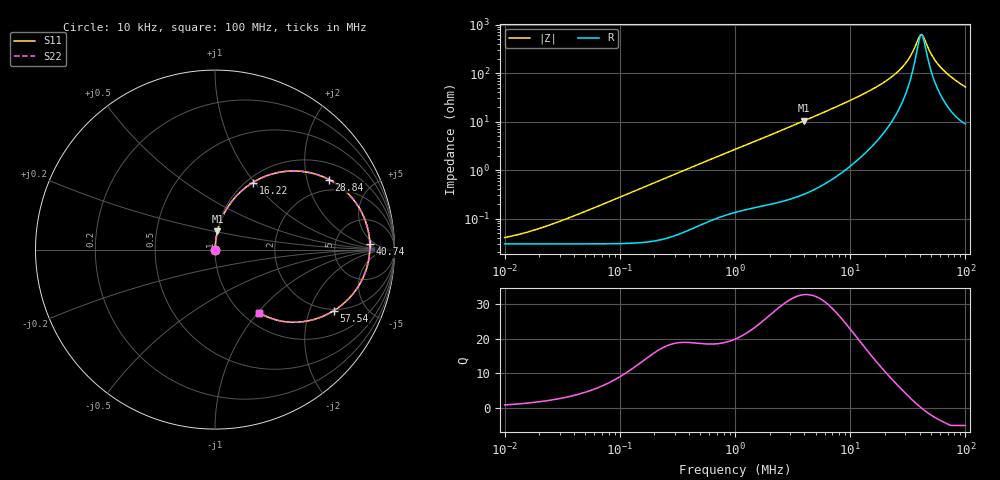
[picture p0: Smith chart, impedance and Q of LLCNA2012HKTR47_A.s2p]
! LLCNA2012HKTR47_A  S-PARAMETER MODEL  ( Standard Model )
! Model Generated by TAIYO YUDEN Corporation (http://www.ty-top.com)
! Version 2.0
! TAIYO YUDEN Control No. 171005
! Copyright(c) 2016 TAIYO YUDEN CO.,LTD. All Rights Reserved.
! Product Description (link to TY-COMPAS)
! https://ds.yuden.co.jp/TYCOMPAS/or/detail?pn=LLCNA2012HKTR47MA&u=M
! Products Name : Inductors
! Characteristics :
!  Inductance : 0.47 [uH] , SRF(min) : - [Hz] , DC Resistance(max) : 36 [mOhm]
!  Rated Current : Saturation  3.21 [A] (dL = 30 [%]), Temp Rise  3.15 [A] (dT = 40 [degC])
!  Case Size : 2.0 x 1.25 / 0.079 x 0.049 [mm/inch] , Thickness : 0.8 / 0.031 [mm/inch]
!  (Conditions: Temperature = 25 [degC] , DC Bias Current = 0 [A])
! External Node Assignments :
!  1  o---GGG---o  2
! GND o---------o GND
! Frequency Range : 10kHz  -  100MHz  [ 402 STEP ]
# MHz S RI R 50
! Freq[MHz].  S11 Real  S11 Imag  S21 Real  S21 Imag  S12 Real  S12 Imag  S22 Real  S22 Imag
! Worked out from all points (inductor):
!   401 points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, 10 kHz to 100 MHz, reference 50 ohm
!   read as one part in series: L = 436 nH near 33.11 kHz
!   highest Q = 32.7 at 3.981 MHz (marker M1), where L = 416 nH
!   self-resonance near 41.59 MHz
!   S11 on the Smith chart (normalised r, x): 10 kHz: 1.00, +0.00; 16.22 MHz: 1.07, +0.98; 28.84 MHz: 1.55, +2.73; 40.74 MHz: 13, +3; 57.54 MHz: 1.93, -2.95; 100 MHz: 1.18, -1.02
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0.01  0.0003 0.000274  0.9997 -0.000274  0.9997 -0.000274  0.0003 0.000274
0.019498  0.0003 0.000534  0.9997 -0.000534  0.9997 -0.000534  0.0003 0.000534
0.046774  0.000302 0.00128  0.9997 -0.00128  0.9997 -0.00128  0.000302 0.00128
0.218776  0.000395 0.00602  0.9996 -0.00602  0.9996 -0.00602  0.000395 0.00602
1  0.00204 0.0265  0.998 -0.0265  0.998 -0.0265  0.00204 0.0265
3.981072  0.0138 0.1022  0.9862 -0.1022  0.9862 -0.1022  0.0138 0.1022
4.677351  0.0184 0.1198  0.9816 -0.1198  0.9816 -0.1198  0.0184 0.1198
10  0.0791 0.2488  0.9209 -0.2488  0.9209 -0.2488  0.0791 0.2488
16.2181  0.2106 0.3737  0.7894 -0.3737  0.7894 -0.3737  0.2106 0.3737
21.87762  0.3855 0.435  0.6145 -0.435  0.6145 -0.435  0.3855 0.435
25.11886  0.5016 0.4335  0.4984 -0.4335  0.4984 -0.4335  0.5016 0.4335
28.84032  0.6348 0.3905  0.3652 -0.3905  0.3652 -0.3905  0.6348 0.3905
33.88442  0.7822 0.2646  0.2178 -0.2646  0.2178 -0.2646  0.7822 0.2646
38.90451  0.8561 0.0933  0.1439 -0.0933  0.1439 -0.0933  0.8561 0.0933
40.73803  0.8629 0.0292  0.1371 -0.0292  0.1371 -0.0292  0.8629 0.0292
41.68694  0.8625 -0.00306  0.1375 0.00306  0.1375 0.00306  0.8625 -0.00306
43.65158  0.8544 -0.0665  0.1456 0.0665  0.1456 0.0665  0.8544 -0.0665
50.11872  0.78 -0.2322  0.22 0.2322  0.22 0.2322  0.78 -0.2322
57.54399  0.6614 -0.3407  0.3386 0.3407  0.3386 0.3407  0.6614 -0.3407
72.4436  0.4548 -0.4045  0.5452 0.4045  0.5452 0.4045  0.4548 -0.4045
87.09636  0.3209 -0.386  0.6791 0.386  0.6791 0.386  0.3209 -0.386
100  0.2468 -0.3519  0.7532 0.3519  0.7532 0.3519  0.2468 -0.3519
